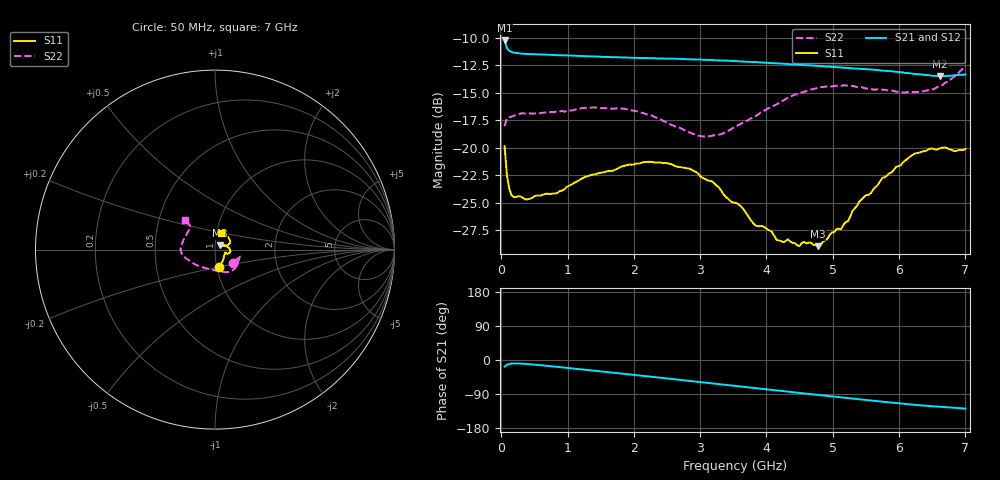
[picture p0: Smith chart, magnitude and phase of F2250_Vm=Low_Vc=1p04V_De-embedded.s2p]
! Integrated Device Technology
! Corporate Headquarters
! 6024 Silver Creek Valley Road
! San Jose, CA 95138  USA
! Phone:  1-408-284-8200
! Toll Free:  1-800-223-1366
! Webpage:  http://www.idt.com/
! Timing and RF Division
! 515 Groton Road, Suite 102
! Westford, MA 01886-6024
! Device:  F2250
! Description: Voltage Variable RF Attenuator
! Frequency:  50.0 -  6000.00 MHz
! Package:  3x3 mm Thin QFN Plastic Package: 16 pin
! Ports:  2 RF, 3 DC
!  Pin  1  = GND
!  Pin  2  = NC
!  Pin  3  = RF1  = Port 1
!  Pin  4  = NC
!  Pin  5  = GND
!  Pin  6  = GND
!  Pin  7  = GND
!  Pin  8  = GND
!  Pin  9  = NC
!  Pin 10  = RF2  = Port 2
!  Pin 11  = NC
!  Pin 12  = GND
!  Pin 13  = GND
!  Pin 14  = VCNTRL
!  Pin 15  = VDD
!  Pin 16  = VMODE
! Vcntrl:  1.040 Volts
! Vmode:  +0.000 Volts
! Vdd:  +3.30  Volts
! Current:  1.190 mA
! Data:  The device was measured on a the F2250 evaluation board which has
!  individual transmission lines to the RF pins.  Data was collected
!  using a calibrated network analyzer.  The evaluation board was
!  de-embedded using a TRL calibration technique.
!  The reference plane is the edge of the package pin.
! Misc:  SN 10
!  Action Tracker AT0258
! Date Measured:  2014-11-26
! Date:  2015-10-15  MJV
! Note:
!  Integrated Device Technology supplies this data as a sample of measured
!  data at the package pin for this product.  Your particular data for this
!  product may vary.
!  Data was taken at 25 degrees C.
!  Integrated Device Technology reserves the right to change this data at anytime.
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# GHz S dB R 50
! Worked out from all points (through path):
!   201 points, 50 MHz to 7 GHz, reference 50 ohm
!   highest |S21| = -10.22 dB at 50 MHz (marker M1); lowest = -13.5 dB at 6.618 GHz (marker M2)
!   group delay of S21, straight-line fit = 50.9 ps
!   lowest |S11| = -29.0 dB at 4.776 GHz (marker M3), VSWR 1.07, Z = 52.6 + j2.6 ohm
!   |S11| at or under -10 dB: start of sweep to end of sweep
!   |S22| runs from -19.0 to -12.6 dB; largest |S21 - S12| = 0.00083
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0.05  -19.85 -76.4  -10.22 -17.4  -10.22 -17.4  -18.01 -35.8
0.08475  -22.52 -53.3  -10.93 -12.4  -10.93 -12.4  -17.28 -20.1
0.1195  -23.70 -41.8  -11.15 -10.3  -11.16 -10.3  -17.20 -15.4
0.189  -24.50 -29.0  -11.33 -9.1  -11.33 -9.1  -17.07 -13.6
0.8145  -24.16 -16.7  -11.55 -17.6  -11.56 -17.6  -16.71 -29.1
1.2315  -22.76 -18.3  -11.65 -25.1  -11.66 -25.1  -16.37 -40.6
1.857  -21.63 -12.6  -11.76 -36.6  -11.75 -36.6  -16.44 -54.2
2.37825  -21.33 -4.5  -11.86 -46.3  -11.86 -46.3  -17.32 -67.1
2.86475  -21.96 6.3  -11.94 -55.6  -11.95 -55.6  -18.65 -88.3
3.0385  -22.74 10.3  -11.98 -58.9  -11.97 -59.0  -18.96 -98.7
3.525  -24.99 23.3  -12.09 -68.3  -12.11 -68.3  -18.08 -129.3
3.83775  -27.08 34.7  -12.19 -74.3  -12.19 -74.3  -17.11 -145.1
4.081  -27.64 44.7  -12.29 -78.9  -12.29 -78.9  -16.27 -155.6
4.1505  -28.37 46.4  -12.31 -80.2  -12.31 -80.2  -16.03 -158.0
4.7065  -28.82 46.4  -12.51 -90.8  -12.51 -90.8  -14.66 -172.8
4.776  -28.95 43.9  -12.54 -92.1  -12.53 -92.1  -14.50 -174.3
5.1235  -27.41 31.6  -12.68 -98.6  -12.67 -98.6  -14.35 178.0
5.4015  -24.88 23.0  -12.80 -103.7  -12.80 -103.7  -14.47 171.6
5.85325  -22.32 20.0  -13.01 -111.8  -13.01 -111.9  -14.79 160.3
6.2355  -20.52 26.3  -13.27 -118.2  -13.26 -118.3  -14.93 147.7
6.61775  -20.04 40.8  -13.47 -123.3  -13.47 -123.3  -14.39 137.1
7  -20.10 70.8  -13.31 -128.4  -13.31 -128.5  -12.55 135.9
